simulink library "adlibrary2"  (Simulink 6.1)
undefined symbols (not defined in the file or in its folder): adlibrary2, ADM, Bit, Black, Box, d2sram_config, DDR, ddr32_config, ddr32xp_config, Generation, II, Inactive, Location, Lower, SDRAM, Simulation, Subsystem, Width, xbsIndex_r3, XPL, XRC, XRM, zbt32_config, zbt64_config, zbtXRC4_config
libraries: xbsIndex_r3 x786
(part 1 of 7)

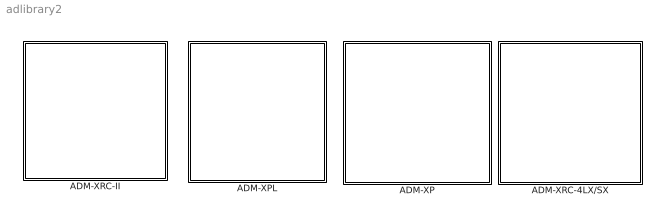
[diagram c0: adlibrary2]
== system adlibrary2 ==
  ADM-XP : Subsystem
  ADM-XPL : Subsystem
  ADM-XRC-4LX/SX : Subsystem  AncestorBlock=adlibrary2/ADM-XRC-II
  ADM-XRC-II : Subsystem

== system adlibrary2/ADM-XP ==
  DDR SDRAM 0 : Subsystem  mask{memsize=1}
      mask prompts: memsize "Simulation RAM Size (Mb)"
  DDR SDRAM 1 : Subsystem  mask{memsize=1}
      mask prompts: memsize "Simulation RAM Size (Mb)"
  DDRII SRAM 0 : Subsystem
  DDRII SRAM 1 : Subsystem
  DDRII SRAM 2 : Subsystem
  DDRII SRAM 3 : Subsystem
  XPL 32 Bit Interface : Subsystem  mask{program='load myprogram.txt', clock_ratio=1.5}
      mask prompts: program "Local Bus Script Program"; clock_ratio "Clock Ratio"
  XPL 64 Bit Interface : Subsystem  mask{program='load myprogram.txt', clock_ratio=1.5}
      mask prompts: program "Local Bus Script Program"; clock_ratio "Clock Ratio"

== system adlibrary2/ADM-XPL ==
  DDR SDRAM : Subsystem  mask{memsize=1}
      mask prompts: memsize "Simulation RAM Size (Mb)"
  XPL 32 Bit Interface : Subsystem  mask{program='load myprogram.txt', clock_ratio=1.5}
      mask prompts: program "Local Bus Script Program"; clock_ratio "Clock Ratio"
  XPL 64 Bit Interface : Subsystem  mask{program='load myprogram.txt', clock_ratio=1.5}
      mask prompts: program "Local Bus Script Program"; clock_ratio "Clock Ratio"
  ZBT SRAM 64 : Subsystem

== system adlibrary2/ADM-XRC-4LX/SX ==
  PLX 32 Bit Interface : Subsystem  mask{program='load myprogram.txt', clock_ratio=1.5}
      mask prompts: program "Local Bus Script Program"; clock_ratio "Clock Ratio"
  ZBT SRAM 0 : Subsystem
  ZBT SRAM 1 : Subsystem
  ZBT SRAM 2 : Subsystem
  ZBT SRAM 3 : Subsystem
  ZBT SRAM 4 : Subsystem
  ZBT SRAM 5 : Subsystem

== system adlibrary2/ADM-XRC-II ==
  PLX 32 Bit Interface : Subsystem  mask{program='load myprogram.txt', clock_ratio=1.5}
      mask prompts: program "Local Bus Script Program"; clock_ratio "Clock Ratio"
  "XRM DDR SDRAM " : Subsystem  mask{memsize=1}
      mask prompts: memsize "Simulation RAM Size (Mb)"
  ZBT SRAM 0 : Subsystem
  ZBT SRAM 1 : Subsystem
  ZBT SRAM 2 : Subsystem
  ZBT SRAM 3 : Subsystem
  ZBT SRAM 4 : Subsystem
  ZBT SRAM 5 : Subsystem

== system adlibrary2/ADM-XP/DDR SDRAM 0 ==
  cache_data_in : Inport  Port=1  LatchInput=off
  cache_addr : Inport  Port=2  LatchInput=off
  cache_write : Inport  Port=3  LatchInput=off
  ddr_page : Inport  Port=4  LatchInput=off
  ddr_addr : Inport  Port=5  LatchInput=off
  ddr_read : Inport  Port=6  LatchInput=off
  ddr_write : Inport  Port=7  LatchInput=off
  adlocb_in : Inport  Port=8  LatchInput=off
  Constant : xbsIndex_r3/Constant  const=0  equ=P=C  arith_type=Unsigned  n_bits=66  bin_pt=0  opselect=C  inp2=PCIN>>17  opr=+  inp1=P  carry=CIN  iostate=0  explicit_period=on  period=1  dbl_ovrd=off
  Convert : xbsIndex_r3/Convert  arith_type=Unsigned  n_bits=66  bin_pt=0  quantization=Truncate  overflow=Wrap  latency=0  explicit_period=on  period=1  dbl_ovrd=off  show_param=off  inserted_by_tool=off  pipeline=off
  DDR SDRAM 32Bit Generation : Subsystem  AncestorBlock=adlibrary2/ADM-XPL/DDR SDRAM /DDR SDRAM 32Bit Generation
  DDR SDRAM 32bit Simulation : Subsystem  mask{memsize=memsize}
      mask prompts: memsize "Simulation Ram Size (Mb)"
  Simulation Multiplexer : xbsIndex_r3/Simulation Multiplexer  sim_sel=1  hw_sel=2
  Simulation Multiplexer1 : xbsIndex_r3/Simulation Multiplexer  sim_sel=1  hw_sel=2
  Simulation Multiplexer2 : xbsIndex_r3/Simulation Multiplexer  sim_sel=1  hw_sel=2
  cache_data_out : Outport
  ddr_busy : Outport  Port=2
  adlocb_out : Outport  Port=3
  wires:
  cache_data_in/1 -> DDR SDRAM 32bit Simulation/1(cache_data_in), DDR SDRAM 32Bit Generation/1(cache_data_in)
  cache_addr/1 -> DDR SDRAM 32bit Simulation/2(cache_addr), DDR SDRAM 32Bit Generation/2(cache_addr)
  cache_write/1 -> DDR SDRAM 32bit Simulation/3(cache_write), DDR SDRAM 32Bit Generation/3(cache_write)
  ddr_page/1 -> DDR SDRAM 32bit Simulation/4(ddr_page), DDR SDRAM 32Bit Generation/4(ddr_page)
  ddr_addr/1 -> DDR SDRAM 32bit Simulation/5(ddr_addr), DDR SDRAM 32Bit Generation/5(ddr_addr)
  ddr_read/1 -> DDR SDRAM 32bit Simulation/6(ddr_read), DDR SDRAM 32Bit Generation/6(ddr_read)
  ddr_write/1 -> DDR SDRAM 32bit Simulation/7(ddr_write), DDR SDRAM 32Bit Generation/7(ddr_write)
  Simulation Multiplexer/1 -> cache_data_out/1
  Simulation Multiplexer1/1 -> ddr_busy/1
  Simulation Multiplexer2/1 -> adlocb_out/1
  DDR SDRAM 32bit Simulation/2(ddr_busy) -> Simulation Multiplexer1/1
  DDR SDRAM 32bit Simulation/1(cache_data_out) -> Simulation Multiplexer/1
  DDR SDRAM 32Bit Generation/1(cache_data_out) -> Simulation Multiplexer/2
  DDR SDRAM 32Bit Generation/2(ddr_busy) -> Simulation Multiplexer1/2
  adlocb_in/1 -> DDR SDRAM 32Bit Generation/8(adlocb_in)
  Constant/1 -> Simulation Multiplexer2/1
  Convert/1 -> Simulation Multiplexer2/2
  DDR SDRAM 32Bit Generation/3(adlocb_out) -> Convert/1

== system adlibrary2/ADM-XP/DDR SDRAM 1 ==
  cache_data_in : Inport  Port=1  LatchInput=off
  cache_addr : Inport  Port=2  LatchInput=off
  cache_write : Inport  Port=3  LatchInput=off
  ddr_page : Inport  Port=4  LatchInput=off
  ddr_addr : Inport  Port=5  LatchInput=off
  ddr_read : Inport  Port=6  LatchInput=off
  ddr_write : Inport  Port=7  LatchInput=off
  adlocb_in : Inport  Port=8  LatchInput=off
  Constant : xbsIndex_r3/Constant  const=0  equ=P=C  arith_type=Unsigned  n_bits=66  bin_pt=0  opselect=C  inp2=PCIN>>17  opr=+  inp1=P  carry=CIN  iostate=0  explicit_period=on  period=1  dbl_ovrd=off
  Convert : xbsIndex_r3/Convert  arith_type=Unsigned  n_bits=66  bin_pt=0  quantization=Truncate  overflow=Wrap  latency=0  explicit_period=on  period=1  dbl_ovrd=off  show_param=off  inserted_by_tool=off  pipeline=off
  DDR SDRAM 32Bit Generation : Subsystem  AncestorBlock=adlibrary2/ADM-XPL/DDR SDRAM /DDR SDRAM 32Bit Generation
  DDR SDRAM 32bit Simulation : Subsystem  mask{memsize=memsize}
      mask prompts: memsize "Simulation Ram Size (Mb)"
  Simulation Multiplexer : xbsIndex_r3/Simulation Multiplexer  sim_sel=1  hw_sel=2
  Simulation Multiplexer1 : xbsIndex_r3/Simulation Multiplexer  sim_sel=1  hw_sel=2
  Simulation Multiplexer2 : xbsIndex_r3/Simulation Multiplexer  sim_sel=1  hw_sel=2
  cache_data_out : Outport
  ddr_busy : Outport  Port=2
  adlocb_out : Outport  Port=3
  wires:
  DDR SDRAM 32Bit Generation/3(adlocb_out) -> Convert/1
  Convert/1 -> Simulation Multiplexer2/2
  Constant/1 -> Simulation Multiplexer2/1
  adlocb_in/1 -> DDR SDRAM 32Bit Generation/8(adlocb_in)
  DDR SDRAM 32Bit Generation/2(ddr_busy) -> Simulation Multiplexer1/2
  DDR SDRAM 32Bit Generation/1(cache_data_out) -> Simulation Multiplexer/2
  DDR SDRAM 32bit Simulation/1(cache_data_out) -> Simulation Multiplexer/1
  DDR SDRAM 32bit Simulation/2(ddr_busy) -> Simulation Multiplexer1/1
  Simulation Multiplexer2/1 -> adlocb_out/1
  Simulation Multiplexer1/1 -> ddr_busy/1
  Simulation Multiplexer/1 -> cache_data_out/1
  ddr_write/1 -> DDR SDRAM 32Bit Generation/7(ddr_write), DDR SDRAM 32bit Simulation/7(ddr_write)
  ddr_read/1 -> DDR SDRAM 32Bit Generation/6(ddr_read), DDR SDRAM 32bit Simulation/6(ddr_read)
  ddr_addr/1 -> DDR SDRAM 32Bit Generation/5(ddr_addr), DDR SDRAM 32bit Simulation/5(ddr_addr)
  ddr_page/1 -> DDR SDRAM 32Bit Generation/4(ddr_page), DDR SDRAM 32bit Simulation/4(ddr_page)
  cache_write/1 -> DDR SDRAM 32Bit Generation/3(cache_write), DDR SDRAM 32bit Simulation/3(cache_write)
  cache_addr/1 -> DDR SDRAM 32Bit Generation/2(cache_addr), DDR SDRAM 32bit Simulation/2(cache_addr)
  cache_data_in/1 -> DDR SDRAM 32Bit Generation/1(cache_data_in), DDR SDRAM 32bit Simulation/1(cache_data_in)

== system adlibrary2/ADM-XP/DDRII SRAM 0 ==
  d : Inport  Port=1  LatchInput=off
  a : Inport  Port=2  LatchInput=off
  w : Inport  Port=3  LatchInput=off
  r : Inport  Port=4  LatchInput=off
  be : Inport  Port=5  LatchInput=off
  adlocb_in : Inport  Port=6  LatchInput=off
  Constant : xbsIndex_r3/Constant  const=0  equ=P=C  arith_type=Unsigned  n_bits=66  bin_pt=0  opselect=C  inp2=PCIN>>17  opr=+  inp1=P  carry=CIN  iostate=0  explicit_period=on  period=1  dbl_ovrd=off
  DDRII SRAM Generation : Subsystem
  DDRII SRAM Simulation : Subsystem
  Register : xbsIndex_r3/Register  init=0  reg_only_valid=off  explicit_period=on  period=1  rst=off  en=off  out_en=off  dbl_ovrd=off  show_param=off
  Register1 : xbsIndex_r3/Register  init=0  reg_only_valid=off  explicit_period=on  period=1  rst=off  en=off  out_en=off  dbl_ovrd=off  show_param=off
  Simulation Multiplexer : xbsIndex_r3/Simulation Multiplexer  sim_sel=1  hw_sel=2
  Simulation Multiplexer1 : xbsIndex_r3/Simulation Multiplexer  sim_sel=1  hw_sel=2
  Simulation Multiplexer2 : xbsIndex_r3/Simulation Multiplexer  sim_sel=1  hw_sel=2
  q : Outport
  qv : Outport  Port=2
  adlocb_out : Outport  Port=3
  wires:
  be/1 -> DDRII SRAM Generation/5(be), DDRII SRAM Simulation/5(be)
  r/1 -> DDRII SRAM Simulation/4(r), DDRII SRAM Generation/4(r)
  w/1 -> DDRII SRAM Generation/3(w), DDRII SRAM Simulation/3(w)
  a/1 -> DDRII SRAM Generation/2(a), DDRII SRAM Simulation/2(a)
  d/1 -> DDRII SRAM Generation/1(d), DDRII SRAM Simulation/1(d)
  DDRII SRAM Simulation/1(q) -> Simulation Multiplexer/1
  DDRII SRAM Generation/1(q) -> Simulation Multiplexer/2
  Simulation Multiplexer/1 -> Register/1
  DDRII SRAM Generation/2(qv) -> Simulation Multiplexer1/2
  DDRII SRAM Simulation/2(qv) -> Simulation Multiplexer1/1
  DDRII SRAM Generation/3(adlocb_out) -> Simulation Multiplexer2/2
  Constant/1 -> Simulation Multiplexer2/1
  Simulation Multiplexer2/1 -> adlocb_out/1
  adlocb_in/1 -> DDRII SRAM Generation/6(adlocb_in)
  Simulation Multiplexer1/1 -> Register1/1
  Register/1 -> q/1
  Register1/1 -> qv/1

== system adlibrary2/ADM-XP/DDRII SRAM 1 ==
  d : Inport  Port=1  LatchInput=off
  a : Inport  Port=2  LatchInput=off
  w : Inport  Port=3  LatchInput=off
  r : Inport  Port=4  LatchInput=off
  be : Inport  Port=5  LatchInput=off
  adlocb_in : Inport  Port=6  LatchInput=off
  Constant : xbsIndex_r3/Constant  const=0  equ=P=C  arith_type=Unsigned  n_bits=66  bin_pt=0  opselect=C  inp2=PCIN>>17  opr=+  inp1=P  carry=CIN  iostate=0  explicit_period=on  period=1  dbl_ovrd=off
  DDRII SRAM Generation : Subsystem
  DDRII SRAM Simulation : Subsystem
  Register : xbsIndex_r3/Register  init=0  reg_only_valid=off  explicit_period=on  period=1  rst=off  en=off  out_en=off  dbl_ovrd=off  show_param=off
  Register1 : xbsIndex_r3/Register  init=0  reg_only_valid=off  explicit_period=on  period=1  rst=off  en=off  out_en=off  dbl_ovrd=off  show_param=off
  Simulation Multiplexer : xbsIndex_r3/Simulation Multiplexer  sim_sel=1  hw_sel=2
  Simulation Multiplexer1 : xbsIndex_r3/Simulation Multiplexer  sim_sel=1  hw_sel=2
  Simulation Multiplexer2 : xbsIndex_r3/Simulation Multiplexer  sim_sel=1  hw_sel=2
  q : Outport
  qv : Outport  Port=2
  adlocb_out : Outport  Port=3
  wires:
  adlocb_in/1 -> DDRII SRAM Generation/6(adlocb_in)
  Simulation Multiplexer2/1 -> adlocb_out/1
  Constant/1 -> Simulation Multiplexer2/1
  DDRII SRAM Generation/3(adlocb_out) -> Simulation Multiplexer2/2
  DDRII SRAM Simulation/2(qv) -> Simulation Multiplexer1/1
  DDRII SRAM Generation/2(qv) -> Simulation Multiplexer1/2
  Simulation Multiplexer/1 -> Register/1
  DDRII SRAM Generation/1(q) -> Simulation Multiplexer/2
  DDRII SRAM Simulation/1(q) -> Simulation Multiplexer/1
  d/1 -> DDRII SRAM Simulation/1(d), DDRII SRAM Generation/1(d)
  a/1 -> DDRII SRAM Simulation/2(a), DDRII SRAM Generation/2(a)
  w/1 -> DDRII SRAM Simulation/3(w), DDRII SRAM Generation/3(w)
  r/1 -> DDRII SRAM Simulation/4(r), DDRII SRAM Generation/4(r)
  be/1 -> DDRII SRAM Simulation/5(be), DDRII SRAM Generation/5(be)
  Simulation Multiplexer1/1 -> Register1/1
  Register/1 -> q/1
  Register1/1 -> qv/1

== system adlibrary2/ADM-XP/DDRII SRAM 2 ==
  d : Inport  Port=1  LatchInput=off
  a : Inport  Port=2  LatchInput=off
  w : Inport  Port=3  LatchInput=off
  r : Inport  Port=4  LatchInput=off
  be : Inport  Port=5  LatchInput=off
  adlocb_in : Inport  Port=6  LatchInput=off
  Constant : xbsIndex_r3/Constant  const=0  equ=P=C  arith_type=Unsigned  n_bits=66  bin_pt=0  opselect=C  inp2=PCIN>>17  opr=+  inp1=P  carry=CIN  iostate=0  explicit_period=on  period=1  dbl_ovrd=off
  DDRII SRAM Generation : Subsystem
  DDRII SRAM Simulation : Subsystem
  Register : xbsIndex_r3/Register  init=0  reg_only_valid=off  explicit_period=on  period=1  rst=off  en=off  out_en=off  dbl_ovrd=off  show_param=off
  Register1 : xbsIndex_r3/Register  init=0  reg_only_valid=off  explicit_period=on  period=1  rst=off  en=off  out_en=off  dbl_ovrd=off  show_param=off
  Simulation Multiplexer : xbsIndex_r3/Simulation Multiplexer  sim_sel=1  hw_sel=2
  Simulation Multiplexer1 : xbsIndex_r3/Simulation Multiplexer  sim_sel=1  hw_sel=2
  Simulation Multiplexer2 : xbsIndex_r3/Simulation Multiplexer  sim_sel=1  hw_sel=2
  q : Outport
  qv : Outport  Port=2
  adlocb_out : Outport  Port=3
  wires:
  adlocb_in/1 -> DDRII SRAM Generation/6(adlocb_in)
  Simulation Multiplexer2/1 -> adlocb_out/1
  Constant/1 -> Simulation Multiplexer2/1
  DDRII SRAM Generation/3(adlocb_out) -> Simulation Multiplexer2/2
  DDRII SRAM Simulation/2(qv) -> Simulation Multiplexer1/1
  DDRII SRAM Generation/2(qv) -> Simulation Multiplexer1/2
  Simulation Multiplexer/1 -> Register/1
  DDRII SRAM Generation/1(q) -> Simulation Multiplexer/2
  DDRII SRAM Simulation/1(q) -> Simulation Multiplexer/1
  d/1 -> DDRII SRAM Simulation/1(d), DDRII SRAM Generation/1(d)
  a/1 -> DDRII SRAM Simulation/2(a), DDRII SRAM Generation/2(a)
  w/1 -> DDRII SRAM Simulation/3(w), DDRII SRAM Generation/3(w)
  r/1 -> DDRII SRAM Simulation/4(r), DDRII SRAM Generation/4(r)
  be/1 -> DDRII SRAM Simulation/5(be), DDRII SRAM Generation/5(be)
  Simulation Multiplexer1/1 -> Register1/1
  Register/1 -> q/1
  Register1/1 -> qv/1

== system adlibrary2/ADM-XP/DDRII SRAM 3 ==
  d : Inport  Port=1  LatchInput=off
  a : Inport  Port=2  LatchInput=off
  w : Inport  Port=3  LatchInput=off
  r : Inport  Port=4  LatchInput=off
  be : Inport  Port=5  LatchInput=off
  adlocb_in : Inport  Port=6  LatchInput=off
  Constant : xbsIndex_r3/Constant  const=0  equ=P=C  arith_type=Unsigned  n_bits=66  bin_pt=0  opselect=C  inp2=PCIN>>17  opr=+  inp1=P  carry=CIN  iostate=0  explicit_period=on  period=1  dbl_ovrd=off
  DDRII SRAM Generation : Subsystem
  DDRII SRAM Simulation : Subsystem
  Register : xbsIndex_r3/Register  init=0  reg_only_valid=off  explicit_period=on  period=1  rst=off  en=off  out_en=off  dbl_ovrd=off  show_param=off
  Register1 : xbsIndex_r3/Register  init=0  reg_only_valid=off  explicit_period=on  period=1  rst=off  en=off  out_en=off  dbl_ovrd=off  show_param=off
  Simulation Multiplexer : xbsIndex_r3/Simulation Multiplexer  sim_sel=1  hw_sel=2
  Simulation Multiplexer1 : xbsIndex_r3/Simulation Multiplexer  sim_sel=1  hw_sel=2
  Simulation Multiplexer2 : xbsIndex_r3/Simulation Multiplexer  sim_sel=1  hw_sel=2
  q : Outport
  qv : Outport  Port=2
  adlocb_out : Outport  Port=3
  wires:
  adlocb_in/1 -> DDRII SRAM Generation/6(adlocb_in)
  Simulation Multiplexer2/1 -> adlocb_out/1
  Constant/1 -> Simulation Multiplexer2/1
  DDRII SRAM Generation/3(adlocb_out) -> Simulation Multiplexer2/2
  DDRII SRAM Simulation/2(qv) -> Simulation Multiplexer1/1
  DDRII SRAM Generation/2(read_pending) -> Simulation Multiplexer1/2
  Simulation Multiplexer/1 -> Register/1
  DDRII SRAM Generation/1(q) -> Simulation Multiplexer/2
  DDRII SRAM Simulation/1(q) -> Simulation Multiplexer/1
  d/1 -> DDRII SRAM Simulation/1(d), DDRII SRAM Generation/1(d)
  a/1 -> DDRII SRAM Simulation/2(a), DDRII SRAM Generation/2(a)
  w/1 -> DDRII SRAM Simulation/3(w), DDRII SRAM Generation/3(w)
  r/1 -> DDRII SRAM Simulation/4(r), DDRII SRAM Generation/4(r)
  be/1 -> DDRII SRAM Simulation/5(be), DDRII SRAM Generation/5(be)
  Simulation Multiplexer1/1 -> Register1/1
  Register/1 -> q/1
  Register1/1 -> qv/1

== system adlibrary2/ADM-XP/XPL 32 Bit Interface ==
  Data_Read : Inport  Port=1  LatchInput=off
  Ack : Inport  Port=2  LatchInput=off
  Status : Inport  Port=3  LatchInput=off
  Read IFIFO : Inport  Port=4  LatchInput=off
  Write OFIFO : Inport  Port=5  LatchInput=off
  OFIFO_Data : Inport  Port=6  LatchInput=off
  ADLOCB_IN : Inport  Port=7  LatchInput=off
  Constant : xbsIndex_r3/Constant  const=0  equ=P=C  arith_type=Unsigned  n_bits=66  bin_pt=0  opselect=C  inp2=PCIN>>17  opr=+  inp1=P  carry=CIN  iostate=0  explicit_period=on  period=1  dbl_ovrd=off
  Convert : xbsIndex_r3/Convert  arith_type=Unsigned  n_bits=66  bin_pt=0  quantization=Truncate  overflow=Wrap  latency=0  explicit_period=on  period=1  dbl_ovrd=off  show_param=off  inserted_by_tool=off  pipeline=off
  Simulation Multiplexer{,1..8,10} (10 alike) : xbsIndex_r3/Simulation Multiplexer  sim_sel=1  hw_sel=2
  XPL 32Bit Generation : Subsystem
  XPL 32Bit Simulation : Subsystem  mask{program=program, clock_ratio=clock_ratio}
      mask prompts: program "Local Bus Script Program"; clock_ratio "Clock Ratio"
  Data_Write : Outport
  Addr : Outport  Port=2
  BE : Outport  Port=3
  Write : Outport  Port=4
  Read : Outport  Port=5
  Control : Outport  Port=6
  IFIFO_Data : Outport  Port=7
  IFIFO_Empty : Outport  Port=8
  OFIFO_Full : Outport  Port=9
  ADLOCB_OUT : Outport  Port=10
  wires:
  ADLOCB_IN/1 -> XPL 32Bit Generation/7(adlocb_in)
  XPL 32Bit Generation/10(adlocb_out) -> Convert/1
  Convert/1 -> Simulation Multiplexer10/2
  Constant/1 -> Simulation Multiplexer10/1
  Simulation Multiplexer10/1 -> ADLOCB_OUT/1
  XPL 32Bit Generation/3(BE) -> Simulation Multiplexer1/2
  XPL 32Bit Simulation/3(BE) -> Simulation Multiplexer1/1
  XPL 32Bit Simulation/2(Addr) -> Simulation Multiplexer8/1
  Simulation Multiplexer8/1 -> Addr/1
  XPL 32Bit Simulation/4(Write) -> Simulation Multiplexer2/1
  XPL 32Bit Simulation/5(Read) -> Simulation Multiplexer3/1
  XPL 32Bit Simulation/6(Control) -> Simulation Multiplexer4/1
  XPL 32Bit Simulation/7(IFIFO_Data) -> Simulation Multiplexer5/1
  XPL 32Bit Simulation/8(IFIFO_Empty) -> Simulation Multiplexer6/1
  Simulation Multiplexer/1 -> Data_Write/1
  Simulation Multiplexer1/1 -> BE/1
  Simulation Multiplexer2/1 -> Write/1
  Simulation Multiplexer3/1 -> Read/1
  Simulation Multiplexer4/1 -> Control/1
  Simulation Multiplexer5/1 -> IFIFO_Data/1
  Simulation Multiplexer6/1 -> IFIFO_Empty/1
  Simulation Multiplexer7/1 -> OFIFO_Full/1
  XPL 32Bit Generation/9(OFIFO_Full) -> Simulation Multiplexer7/2
  XPL 32Bit Generation/8(IFIFO_Empty) -> Simulation Multiplexer6/2
  XPL 32Bit Generation/7(IFIFO_Data) -> Simulation Multiplexer5/2
  XPL 32Bit Generation/6(Control) -> Simulation Multiplexer4/2
  XPL 32Bit Generation/5(Read) -> Simulation Multiplexer3/2
  XPL 32Bit Generation/4(Write) -> Simulation Multiplexer2/2
  XPL 32Bit Generation/2(Addr) -> Simulation Multiplexer8/2
  XPL 32Bit Generation/1(Data_Write) -> Simulation Multiplexer/2
  XPL 32Bit Simulation/1(Data_Write) -> Simulation Multiplexer/1
  XPL 32Bit Simulation/9(OFIFO_Full) -> Simulation Multiplexer7/1
  Data_Read/1 -> XPL 32Bit Simulation/1(Data_Read), XPL 32Bit Generation/1(Data_Read)
  Ack/1 -> XPL 32Bit Simulation/2(Ack), XPL 32Bit Generation/2(Ack)
  Status/1 -> XPL 32Bit Simulation/3(Status), XPL 32Bit Generation/3(Status)
  Read IFIFO/1 -> XPL 32Bit Simulation/4(Read IFIFO), XPL 32Bit Generation/4(Read IFIFO)
  Write OFIFO/1 -> XPL 32Bit Simulation/5(Write OFIFO), XPL 32Bit Generation/5(Write OFIFO)
  OFIFO_Data/1 -> XPL 32Bit Simulation/6(OFIFO_Data), XPL 32Bit Generation/6(OFIFO_Data)

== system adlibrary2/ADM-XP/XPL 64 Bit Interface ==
  Data_Read : Inport  Port=1  LatchInput=off
  Ack : Inport  Port=2  LatchInput=off
  Status : Inport  Port=3  LatchInput=off
  Read IFIFO : Inport  Port=4  LatchInput=off
  Write OFIFO : Inport  Port=5  LatchInput=off
  OFIFO_Data : Inport  Port=6  LatchInput=off
  ADLOCB_IN : Inport  Port=7  LatchInput=off
  Constant : xbsIndex_r3/Constant  const=0  equ=P=C  arith_type=Unsigned  n_bits=66  bin_pt=0  opselect=C  inp2=PCIN>>17  opr=+  inp1=P  carry=CIN  iostate=0  explicit_period=on  period=1  dbl_ovrd=off
  Convert : xbsIndex_r3/Convert  arith_type=Unsigned  n_bits=66  bin_pt=0  quantization=Truncate  overflow=Wrap  latency=0  explicit_period=on  period=1  dbl_ovrd=off  show_param=off  inserted_by_tool=off  pipeline=off
  Simulation Multiplexer{,1..9} (10 alike) : xbsIndex_r3/Simulation Multiplexer  sim_sel=1  hw_sel=2
  XPL 64Bit Generation : Subsystem
  XPL 64Bit Simulation : Subsystem  mask{program=program, clock_ratio=clock_ratio}
      mask prompts: program "Local Bus Script Program"; clock_ratio "Clock Ratio"
  Data_Write : Outport
  Addr : Outport  Port=2
  BE : Outport  Port=3
  Write : Outport  Port=4
  Read : Outport  Port=5
  Control : Outport  Port=6
  IFIFO_Data : Outport  Port=7
  IFIFO_Empty : Outport  Port=8
  OFIFO_Full : Outport  Port=9
  ADLOCB_OUT : Outport  Port=10
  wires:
  XPL 64Bit Generation/10(adlocb_out) -> Convert/1
  Convert/1 -> Simulation Multiplexer9/2
  Constant/1 -> Simulation Multiplexer9/1
  ADLOCB_IN/1 -> XPL 64Bit Generation/7(adlocb_in)
  Simulation Multiplexer9/1 -> ADLOCB_OUT/1
  XPL 64Bit Simulation/3(BE) -> Simulation Multiplexer8/1
  XPL 64Bit Generation/3(BE) -> Simulation Multiplexer8/2
  Simulation Multiplexer8/1 -> BE/1
  OFIFO_Data/1 -> XPL 64Bit Generation/6(OFIFO_Data), XPL 64Bit Simulation/6(OFIFO_Data)
  Write OFIFO/1 -> XPL 64Bit Generation/5(Write OFIFO), XPL 64Bit Simulation/5(Write OFIFO)
  Read IFIFO/1 -> XPL 64Bit Generation/4(Read IFIFO), XPL 64Bit Simulation/4(Read IFIFO)
  Status/1 -> XPL 64Bit Generation/3(Status), XPL 64Bit Simulation/3(Status)
  Ack/1 -> XPL 64Bit Generation/2(Ack), XPL 64Bit Simulation/2(Ack)
  Data_Read/1 -> XPL 64Bit Generation/1(Data_Read), XPL 64Bit Simulation/1(Data_Read)
  XPL 64Bit Simulation/9(OFIFO_Full) -> Simulation Multiplexer7/1
  XPL 64Bit Simulation/8(IFIFO_Empty) -> Simulation Multiplexer6/1
  XPL 64Bit Simulation/7(IFIFO_Data) -> Simulation Multiplexer5/1
  XPL 64Bit Simulation/6(Control) -> Simulation Multiplexer4/1
  XPL 64Bit Simulation/5(Read) -> Simulation Multiplexer3/1
  XPL 64Bit Simulation/4(Write) -> Simulation Multiplexer2/1
  XPL 64Bit Simulation/2(Addr) -> Simulation Multiplexer1/1
  XPL 64Bit Simulation/1(Data_Write) -> Simulation Multiplexer/1
  XPL 64Bit Generation/1(Data_Write) -> Simulation Multiplexer/2
  XPL 64Bit Generation/2(Addr) -> Simulation Multiplexer1/2
  XPL 64Bit Generation/4(Write) -> Simulation Multiplexer2/2
  XPL 64Bit Generation/5(Read) -> Simulation Multiplexer3/2
  XPL 64Bit Generation/6(Control) -> Simulation Multiplexer4/2
  XPL 64Bit Generation/7(IFIFO_Data) -> Simulation Multiplexer5/2
  XPL 64Bit Generation/8(IFIFO_Empty) -> Simulation Multiplexer6/2
  XPL 64Bit Generation/9(OFIFO_Full) -> Simulation Multiplexer7/2
  Simulation Multiplexer7/1 -> OFIFO_Full/1
  Simulation Multiplexer6/1 -> IFIFO_Empty/1
  Simulation Multiplexer5/1 -> IFIFO_Data/1
  Simulation Multiplexer4/1 -> Control/1
  Simulation Multiplexer3/1 -> Read/1
  Simulation Multiplexer2/1 -> Write/1
  Simulation Multiplexer1/1 -> Addr/1
  Simulation Multiplexer/1 -> Data_Write/1

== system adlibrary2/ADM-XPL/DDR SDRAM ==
  cache_data_in : Inport  Port=1  LatchInput=off
  cache_addr : Inport  Port=2  LatchInput=off
  cache_write : Inport  Port=3  LatchInput=off
  ddr_page : Inport  Port=4  LatchInput=off
  ddr_addr : Inport  Port=5  LatchInput=off
  ddr_read : Inport  Port=6  LatchInput=off
  ddr_write : Inport  Port=7  LatchInput=off
  adlocb_in : Inport  Port=8  LatchInput=off
  Constant : xbsIndex_r3/Constant  const=0  equ=P=C  arith_type=Unsigned  n_bits=66  bin_pt=0  opselect=C  inp2=PCIN>>17  opr=+  inp1=P  carry=CIN  iostate=0  explicit_period=on  period=1  dbl_ovrd=off
  Convert : xbsIndex_r3/Convert  arith_type=Unsigned  n_bits=66  bin_pt=0  quantization=Truncate  overflow=Wrap  latency=0  explicit_period=on  period=1  dbl_ovrd=off  show_param=off  inserted_by_tool=off  pipeline=off
  DDR SDRAM 32Bit Generation : Subsystem  AncestorBlock=adlibrary2/ADM-XPL/DDR SDRAM /DDR SDRAM 32Bit Generation
  DDR SDRAM 32bit Simulation : Subsystem  mask{memsize=memsize}
      mask prompts: memsize "Simulation Ram Size (Mb)"
  Simulation Multiplexer : xbsIndex_r3/Simulation Multiplexer  sim_sel=1  hw_sel=2
  Simulation Multiplexer1 : xbsIndex_r3/Simulation Multiplexer  sim_sel=1  hw_sel=2
  Simulation Multiplexer2 : xbsIndex_r3/Simulation Multiplexer  sim_sel=1  hw_sel=2
  cache_data_out : Outport
  ddr_busy : Outport  Port=2
  adlocb_out : Outport  Port=3
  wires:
  DDR SDRAM 32Bit Generation/3(adlocb_out) -> Convert/1
  Convert/1 -> Simulation Multiplexer2/2
  Constant/1 -> Simulation Multiplexer2/1
  adlocb_in/1 -> DDR SDRAM 32Bit Generation/8(adlocb_in)
  DDR SDRAM 32Bit Generation/2(ddr_busy) -> Simulation Multiplexer1/2
  DDR SDRAM 32Bit Generation/1(cache_data_out) -> Simulation Multiplexer/2
  DDR SDRAM 32bit Simulation/1(cache_data_out) -> Simulation Multiplexer/1
  DDR SDRAM 32bit Simulation/2(ddr_busy) -> Simulation Multiplexer1/1
  Simulation Multiplexer2/1 -> adlocb_out/1
  Simulation Multiplexer1/1 -> ddr_busy/1
  Simulation Multiplexer/1 -> cache_data_out/1
  ddr_write/1 -> DDR SDRAM 32Bit Generation/7(ddr_write), DDR SDRAM 32bit Simulation/7(ddr_write)
  ddr_read/1 -> DDR SDRAM 32Bit Generation/6(ddr_read), DDR SDRAM 32bit Simulation/6(ddr_read)
  ddr_addr/1 -> DDR SDRAM 32Bit Generation/5(ddr_addr), DDR SDRAM 32bit Simulation/5(ddr_addr)
  ddr_page/1 -> DDR SDRAM 32Bit Generation/4(ddr_page), DDR SDRAM 32bit Simulation/4(ddr_page)
  cache_write/1 -> DDR SDRAM 32Bit Generation/3(cache_write), DDR SDRAM 32bit Simulation/3(cache_write)
  cache_addr/1 -> DDR SDRAM 32Bit Generation/2(cache_addr), DDR SDRAM 32bit Simulation/2(cache_addr)
  cache_data_in/1 -> DDR SDRAM 32Bit Generation/1(cache_data_in), DDR SDRAM 32bit Simulation/1(cache_data_in)

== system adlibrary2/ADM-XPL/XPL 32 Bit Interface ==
  Data_Read : Inport  Port=1  LatchInput=off
  Ack : Inport  Port=2  LatchInput=off
  Status : Inport  Port=3  LatchInput=off
  Read IFIFO : Inport  Port=4  LatchInput=off
  Write OFIFO : Inport  Port=5  LatchInput=off
  OFIFO_Data : Inport  Port=6  LatchInput=off
  ADLOCB_IN : Inport  Port=7  LatchInput=off
  Constant : xbsIndex_r3/Constant  const=0  equ=P=C  arith_type=Unsigned  n_bits=66  bin_pt=0  opselect=C  inp2=PCIN>>17  opr=+  inp1=P  carry=CIN  iostate=0  explicit_period=on  period=1  dbl_ovrd=off
  Convert : xbsIndex_r3/Convert  arith_type=Unsigned  n_bits=66  bin_pt=0  quantization=Truncate  overflow=Wrap  latency=0  explicit_period=on  period=1  dbl_ovrd=off  show_param=off  inserted_by_tool=off  pipeline=off
  Simulation Multiplexer{,1..8,10} (10 alike) : xbsIndex_r3/Simulation Multiplexer  sim_sel=1  hw_sel=2
  XPL 32Bit Generation : Subsystem
  XPL 32Bit Simulation : Subsystem  mask{program=program, clock_ratio=clock_ratio}
      mask prompts: program "Local Bus Script Program"; clock_ratio "Clock Ratio"
  Data_Write : Outport
  Addr : Outport  Port=2
  BE : Outport  Port=3
  Write : Outport  Port=4
  Read : Outport  Port=5
  Control : Outport  Port=6
  IFIFO_Data : Outport  Port=7
  IFIFO_Empty : Outport  Port=8
  OFIFO_Full : Outport  Port=9
  ADLOCB_OUT : Outport  Port=10
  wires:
  OFIFO_Data/1 -> XPL 32Bit Generation/6(OFIFO_Data), XPL 32Bit Simulation/6(OFIFO_Data)
  Write OFIFO/1 -> XPL 32Bit Generation/5(Write OFIFO), XPL 32Bit Simulation/5(Write OFIFO)
  Read IFIFO/1 -> XPL 32Bit Generation/4(Read IFIFO), XPL 32Bit Simulation/4(Read IFIFO)
  Status/1 -> XPL 32Bit Generation/3(Status), XPL 32Bit Simulation/3(Status)
  Ack/1 -> XPL 32Bit Generation/2(Ack), XPL 32Bit Simulation/2(Ack)
  Data_Read/1 -> XPL 32Bit Generation/1(Data_Read), XPL 32Bit Simulation/1(Data_Read)
  XPL 32Bit Simulation/9(OFIFO_Full) -> Simulation Multiplexer7/1
  XPL 32Bit Simulation/1(Data_Write) -> Simulation Multiplexer/1
  XPL 32Bit Generation/1(Data_Write) -> Simulation Multiplexer/2
  XPL 32Bit Generation/2(Addr) -> Simulation Multiplexer8/2
  XPL 32Bit Generation/4(Write) -> Simulation Multiplexer2/2
  XPL 32Bit Generation/5(Read) -> Simulation Multiplexer3/2
  XPL 32Bit Generation/6(Control) -> Simulation Multiplexer4/2
  XPL 32Bit Generation/7(IFIFO_Data) -> Simulation Multiplexer5/2
  XPL 32Bit Generation/8(IFIFO_Empty) -> Simulation Multiplexer6/2
  XPL 32Bit Generation/9(OFIFO_Full) -> Simulation Multiplexer7/2
  Simulation Multiplexer7/1 -> OFIFO_Full/1
  Simulation Multiplexer6/1 -> IFIFO_Empty/1
  Simulation Multiplexer5/1 -> IFIFO_Data/1
  Simulation Multiplexer4/1 -> Control/1
  Simulation Multiplexer3/1 -> Read/1
  Simulation Multiplexer2/1 -> Write/1
  Simulation Multiplexer1/1 -> BE/1
  Simulation Multiplexer/1 -> Data_Write/1
  XPL 32Bit Simulation/8(IFIFO_Empty) -> Simulation Multiplexer6/1
  XPL 32Bit Simulation/7(IFIFO_Data) -> Simulation Multiplexer5/1
  XPL 32Bit Simulation/6(Control) -> Simulation Multiplexer4/1
  XPL 32Bit Simulation/5(Read) -> Simulation Multiplexer3/1
  XPL 32Bit Simulation/4(Write) -> Simulation Multiplexer2/1
  Simulation Multiplexer8/1 -> Addr/1
  XPL 32Bit Simulation/2(Addr) -> Simulation Multiplexer8/1
  XPL 32Bit Simulation/3(BE) -> Simulation Multiplexer1/1
  XPL 32Bit Generation/3(BE) -> Simulation Multiplexer1/2
  Simulation Multiplexer10/1 -> ADLOCB_OUT/1
  Constant/1 -> Simulation Multiplexer10/1
  Convert/1 -> Simulation Multiplexer10/2
  XPL 32Bit Generation/10(adlocb_out) -> Convert/1
  ADLOCB_IN/1 -> XPL 32Bit Generation/7(adlocb_in)

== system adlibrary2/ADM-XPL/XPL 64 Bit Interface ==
  Data_Read : Inport  Port=1  LatchInput=off
  Ack : Inport  Port=2  LatchInput=off
  Status : Inport  Port=3  LatchInput=off
  Read IFIFO : Inport  Port=4  LatchInput=off
  Write OFIFO : Inport  Port=5  LatchInput=off
  OFIFO_Data : Inport  Port=6  LatchInput=off
  ADLOCB_IN : Inport  Port=7  LatchInput=off
  Constant : xbsIndex_r3/Constant  const=0  equ=P=C  arith_type=Unsigned  n_bits=66  bin_pt=0  opselect=C  inp2=PCIN>>17  opr=+  inp1=P  carry=CIN  iostate=0  explicit_period=on  period=1  dbl_ovrd=off
  Convert : xbsIndex_r3/Convert  arith_type=Unsigned  n_bits=66  bin_pt=0  quantization=Truncate  overflow=Wrap  latency=0  explicit_period=on  period=1  dbl_ovrd=off  show_param=off  inserted_by_tool=off  pipeline=off
  Simulation Multiplexer{,1..9} (10 alike) : xbsIndex_r3/Simulation Multiplexer  sim_sel=1  hw_sel=2
  XPL 64Bit Generation : Subsystem
  XPL 64Bit Simulation : Subsystem  mask{program=program, clock_ratio=clock_ratio}
      mask prompts: program "Local Bus Script Program"; clock_ratio "Clock Ratio"
  Data_Write : Outport
  Addr : Outport  Port=2
  BE : Outport  Port=3
  Write : Outport  Port=4
  Read : Outport  Port=5
  Control : Outport  Port=6
  IFIFO_Data : Outport  Port=7
  IFIFO_Empty : Outport  Port=8
  OFIFO_Full : Outport  Port=9
  ADLOCB_OUT : Outport  Port=10
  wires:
  Simulation Multiplexer/1 -> Data_Write/1
  Simulation Multiplexer1/1 -> Addr/1
  Simulation Multiplexer2/1 -> Write/1
  Simulation Multiplexer3/1 -> Read/1
  Simulation Multiplexer4/1 -> Control/1
  Simulation Multiplexer5/1 -> IFIFO_Data/1
  Simulation Multiplexer6/1 -> IFIFO_Empty/1
  Simulation Multiplexer7/1 -> OFIFO_Full/1
  XPL 64Bit Generation/9(OFIFO_Full) -> Simulation Multiplexer7/2
  XPL 64Bit Generation/8(IFIFO_Empty) -> Simulation Multiplexer6/2
  XPL 64Bit Generation/7(IFIFO_Data) -> Simulation Multiplexer5/2
  XPL 64Bit Generation/6(Control) -> Simulation Multiplexer4/2
  XPL 64Bit Generation/5(Read) -> Simulation Multiplexer3/2
  XPL 64Bit Generation/4(Write) -> Simulation Multiplexer2/2
  XPL 64Bit Generation/2(Addr) -> Simulation Multiplexer1/2
  XPL 64Bit Generation/1(Data_Write) -> Simulation Multiplexer/2
  XPL 64Bit Simulation/1(Data_Write) -> Simulation Multiplexer/1
  XPL 64Bit Simulation/2(Addr) -> Simulation Multiplexer1/1
  XPL 64Bit Simulation/4(Write) -> Simulation Multiplexer2/1
  XPL 64Bit Simulation/5(Read) -> Simulation Multiplexer3/1
  XPL 64Bit Simulation/6(Control) -> Simulation Multiplexer4/1
  XPL 64Bit Simulation/7(IFIFO_Data) -> Simulation Multiplexer5/1
  XPL 64Bit Simulation/8(IFIFO_Empty) -> Simulation Multiplexer6/1
  XPL 64Bit Simulation/9(OFIFO_Full) -> Simulation Multiplexer7/1
  Data_Read/1 -> XPL 64Bit Simulation/1(Data_Read), XPL 64Bit Generation/1(Data_Read)
  Ack/1 -> XPL 64Bit Simulation/2(Ack), XPL 64Bit Generation/2(Ack)
  Status/1 -> XPL 64Bit Simulation/3(Status), XPL 64Bit Generation/3(Status)
  Read IFIFO/1 -> XPL 64Bit Simulation/4(Read IFIFO), XPL 64Bit Generation/4(Read IFIFO)
  Write OFIFO/1 -> XPL 64Bit Simulation/5(Write OFIFO), XPL 64Bit Generation/5(Write OFIFO)
  OFIFO_Data/1 -> XPL 64Bit Simulation/6(OFIFO_Data), XPL 64Bit Generation/6(OFIFO_Data)
  Simulation Multiplexer8/1 -> BE/1
  XPL 64Bit Generation/3(BE) -> Simulation Multiplexer8/2
  XPL 64Bit Simulation/3(BE) -> Simulation Multiplexer8/1
  Simulation Multiplexer9/1 -> ADLOCB_OUT/1
  ADLOCB_IN/1 -> XPL 64Bit Generation/7(adlocb_in)
  Constant/1 -> Simulation Multiplexer9/1
  Convert/1 -> Simulation Multiplexer9/2
  XPL 64Bit Generation/10(adlocb_out) -> Convert/1

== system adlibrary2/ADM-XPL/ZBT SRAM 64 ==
  d : Inport  Port=1  LatchInput=off
  a : Inport  Port=2  LatchInput=off
  w : Inport  Port=3  LatchInput=off
  r : Inport  Port=4  LatchInput=off
  be : Inport  Port=5  LatchInput=off
  adlocb_in : Inport  Port=6  LatchInput=off
  Constant : xbsIndex_r3/Constant  const=0  equ=P=C  arith_type=Unsigned  n_bits=66  bin_pt=0  opselect=C  inp2=PCIN>>17  opr=+  inp1=P  carry=CIN  iostate=0  explicit_period=on  period=1  dbl_ovrd=off
  Simulation Multiplexer : xbsIndex_r3/Simulation Multiplexer  sim_sel=1  hw_sel=2
  Simulation Multiplexer1 : xbsIndex_r3/Simulation Multiplexer  sim_sel=1  hw_sel=2
  Simulation Multiplexer2 : xbsIndex_r3/Simulation Multiplexer  sim_sel=1  hw_sel=2
  ZBT SRAM 64Bit Generation : Subsystem
  ZBT SRAM 64bit Simulation : Subsystem
  q : Outport
  qv : Outport  Port=2
  adlocb_out : Outport  Port=3
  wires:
  Simulation Multiplexer/1 -> q/1
  ZBT SRAM 64Bit Generation/1(q) -> Simulation Multiplexer/2
  ZBT SRAM 64bit Simulation/1(q) -> Simulation Multiplexer/1
  d/1 -> ZBT SRAM 64bit Simulation/1(d), ZBT SRAM 64Bit Generation/1(d)
  a/1 -> ZBT SRAM 64bit Simulation/2(a), ZBT SRAM 64Bit Generation/2(a)
  w/1 -> ZBT SRAM 64bit Simulation/3(w), ZBT SRAM 64Bit Generation/3(w)
  Simulation Multiplexer1/1 -> qv/1
  r/1 -> ZBT SRAM 64bit Simulation/4(r), ZBT SRAM 64Bit Generation/4(r)
  ZBT SRAM 64bit Simulation/2(qv) -> Simulation Multiplexer1/1
  ZBT SRAM 64Bit Generation/2(qv) -> Simulation Multiplexer1/2
  be/1 -> ZBT SRAM 64bit Simulation/5(be), ZBT SRAM 64Bit Generation/5(be)
  Simulation Multiplexer2/1 -> adlocb_out/1
  ZBT SRAM 64Bit Generation/3(adlocb_out) -> Simulation Multiplexer2/2
  Constant/1 -> Simulation Multiplexer2/1
  adlocb_in/1 -> ZBT SRAM 64Bit Generation/6(adlocb_in)

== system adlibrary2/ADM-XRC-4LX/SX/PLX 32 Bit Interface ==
  Data_Read : Inport  Port=1  LatchInput=off
  Ack : Inport  Port=2  LatchInput=off
  Status : Inport  Port=3  LatchInput=off
  Read IFIFO : Inport  Port=4  LatchInput=off
  Write OFIFO : Inport  Port=5  LatchInput=off
  OFIFO_Data : Inport  Port=6  LatchInput=off
  ADLOCB_IN : Inport  Port=7  LatchInput=off
  Constant : xbsIndex_r3/Constant  const=0  equ=P=C  arith_type=Unsigned  n_bits=34  bin_pt=0  opselect=C  inp2=PCIN>>17  opr=+  inp1=P  carry=CIN  iostate=0  explicit_period=on  period=1  dbl_ovrd=off
  Convert : xbsIndex_r3/Convert  arith_type=Unsigned  n_bits=34  bin_pt=0  quantization=Truncate  overflow=Wrap  latency=0  explicit_period=on  period=1  dbl_ovrd=off  show_param=off  inserted_by_tool=off  pipeline=off
  PLX 32Bit Generation : Subsystem
  PLX 32Bit Simulation : Subsystem  mask{program=program, clock_ratio=clock_ratio}
      mask prompts: program "Local Bus Script Program"; clock_ratio "Clock Ratio"
  Simulation Multiplexer{,1..9} (10 alike) : xbsIndex_r3/Simulation Multiplexer  sim_sel=1  hw_sel=2
  Data_Write : Outport
  Addr : Outport  Port=2
  BE : Outport  Port=3
  Write : Outport  Port=4
  Read : Outport  Port=5
  Control : Outport  Port=6
  IFIFO_Data : Outport  Port=7
  IFIFO_Empty : Outport  Port=8
  OFIFO_Full : Outport  Port=9
  ADLOCB_OUT : Outport  Port=10
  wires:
  Data_Read/1 -> PLX 32Bit Generation/1(Data_Read), PLX 32Bit Simulation/1(Data_Read)
  Ack/1 -> PLX 32Bit Generation/2(Ack), PLX 32Bit Simulation/2(Ack)
  Status/1 -> PLX 32Bit Generation/3(Status), PLX 32Bit Simulation/3(Status)
  Read IFIFO/1 -> PLX 32Bit Generation/4(Read IFIFO), PLX 32Bit Simulation/4(Read IFIFO)
  Write OFIFO/1 -> PLX 32Bit Generation/5(Write OFIFO), PLX 32Bit Simulation/5(Write OFIFO)
  OFIFO_Data/1 -> PLX 32Bit Generation/6(OFIFO_Data), PLX 32Bit Simulation/6(OFIFO_Data)
  Simulation Multiplexer/1 -> Data_Write/1
  Simulation Multiplexer1/1 -> Addr/1
  Simulation Multiplexer2/1 -> Write/1
  Simulation Multiplexer3/1 -> Read/1
  Simulation Multiplexer4/1 -> Control/1
  Simulation Multiplexer5/1 -> IFIFO_Data/1
  Simulation Multiplexer6/1 -> IFIFO_Empty/1
  Simulation Multiplexer7/1 -> OFIFO_Full/1
  PLX 32Bit Generation/9(OFIFO_Full) -> Simulation Multiplexer7/2
  PLX 32Bit Generation/8(IFIFO_Empty) -> Simulation Multiplexer6/2
  PLX 32Bit Generation/7(IFIFO_Data) -> Simulation Multiplexer5/2
  PLX 32Bit Generation/6(Control) -> Simulation Multiplexer4/2
  PLX 32Bit Generation/5(Read) -> Simulation Multiplexer3/2
  PLX 32Bit Generation/4(Write) -> Simulation Multiplexer2/2
  PLX 32Bit Generation/2(Addr) -> Simulation Multiplexer1/2
  PLX 32Bit Generation/1(Data_Write) -> Simulation Multiplexer/2
  PLX 32Bit Simulation/1(Data_Write) -> Simulation Multiplexer/1
  PLX 32Bit Simulation/2(Addr) -> Simulation Multiplexer1/1
  PLX 32Bit Simulation/4(Write) -> Simulation Multiplexer2/1
  PLX 32Bit Simulation/5(Read) -> Simulation Multiplexer3/1
  PLX 32Bit Simulation/6(Control) -> Simulation Multiplexer4/1
  PLX 32Bit Simulation/7(IFIFO_Data) -> Simulation Multiplexer5/1
  PLX 32Bit Simulation/8(IFIFO_Empty) -> Simulation Multiplexer6/1
  PLX 32Bit Simulation/9(OFIFO_Full) -> Simulation Multiplexer7/1
  Simulation Multiplexer8/1 -> BE/1
  PLX 32Bit Generation/3(BE) -> Simulation Multiplexer8/2
  PLX 32Bit Simulation/3(BE) -> Simulation Multiplexer8/1
  Simulation Multiplexer9/1 -> ADLOCB_OUT/1
  PLX 32Bit Generation/10(ADLOCB_OUT) -> Convert/1
  ADLOCB_IN/1 -> PLX 32Bit Generation/7(ADLOCB_IN)
  Constant/1 -> Simulation Multiplexer9/1
  Convert/1 -> Simulation Multiplexer9/2

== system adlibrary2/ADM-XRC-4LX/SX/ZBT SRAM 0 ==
  d : Inport  Port=1  LatchInput=off
  a : Inport  Port=2  LatchInput=off
  w : Inport  Port=3  LatchInput=off
  r : Inport  Port=4  LatchInput=off
  be : Inport  Port=5  LatchInput=off
  adlocb_in : Inport  Port=6  LatchInput=off
  Constant : xbsIndex_r3/Constant  const=0  equ=P=C  arith_type=Unsigned  n_bits=34  bin_pt=0  opselect=C  inp2=PCIN>>17  opr=+  inp1=P  carry=CIN  iostate=0  explicit_period=on  period=1  dbl_ovrd=off
  Simulation Multiplexer : xbsIndex_r3/Simulation Multiplexer  sim_sel=1  hw_sel=2
  Simulation Multiplexer1 : xbsIndex_r3/Simulation Multiplexer  sim_sel=1  hw_sel=2
  Simulation Multiplexer2 : xbsIndex_r3/Simulation Multiplexer  sim_sel=1  hw_sel=2
  ZBT SRAM 32Bit Generation : Subsystem
  ZBT SRAM 32Bit Simulation : Subsystem
  q : Outport
  qv : Outport  Port=2
  adlocb_out : Outport  Port=3
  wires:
  r/1 -> ZBT SRAM 32Bit Generation/4(r), ZBT SRAM 32Bit Simulation/4(r)
  w/1 -> ZBT SRAM 32Bit Generation/3(w), ZBT SRAM 32Bit Simulation/3(w)
  a/1 -> ZBT SRAM 32Bit Generation/2(a), ZBT SRAM 32Bit Simulation/2(a)
  d/1 -> ZBT SRAM 32Bit Generation/1(d), ZBT SRAM 32Bit Simulation/1(d)
  ZBT SRAM 32Bit Simulation/2(qv) -> Simulation Multiplexer1/1
  ZBT SRAM 32Bit Simulation/1(q) -> Simulation Multiplexer/1
  ZBT SRAM 32Bit Generation/1(q) -> Simulation Multiplexer/2
  ZBT SRAM 32Bit Generation/2(qv) -> Simulation Multiplexer1/2
  Simulation Multiplexer1/1 -> qv/1
  Simulation Multiplexer/1 -> q/1
  be/1 -> ZBT SRAM 32Bit Simulation/5(be), ZBT SRAM 32Bit Generation/5(be)
  Simulation Multiplexer2/1 -> adlocb_out/1
  ZBT SRAM 32Bit Generation/3(adlocb_out) -> Simulation Multiplexer2/2
  adlocb_in/1 -> ZBT SRAM 32Bit Generation/6(adlocb_in)
  Constant/1 -> Simulation Multiplexer2/1

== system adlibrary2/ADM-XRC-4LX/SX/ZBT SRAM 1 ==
  d : Inport  Port=1  LatchInput=off
  a : Inport  Port=2  LatchInput=off
  w : Inport  Port=3  LatchInput=off
  r : Inport  Port=4  LatchInput=off
  be : Inport  Port=5  LatchInput=off
  adlocb_in : Inport  Port=6  LatchInput=off
  Constant : xbsIndex_r3/Constant  const=0  equ=P=C  arith_type=Unsigned  n_bits=34  bin_pt=0  opselect=C  inp2=PCIN>>17  opr=+  inp1=P  carry=CIN  iostate=0  explicit_period=on  period=1  dbl_ovrd=off
  Convert : xbsIndex_r3/Convert  arith_type=Unsigned  n_bits=34  bin_pt=0  quantization=Truncate  overflow=Wrap  latency=0  explicit_period=on  period=1  dbl_ovrd=off  show_param=off  inserted_by_tool=off  pipeline=off
  Simulation Multiplexer : xbsIndex_r3/Simulation Multiplexer  sim_sel=1  hw_sel=2
  Simulation Multiplexer1 : xbsIndex_r3/Simulation Multiplexer  sim_sel=1  hw_sel=2
  Simulation Multiplexer2 : xbsIndex_r3/Simulation Multiplexer  sim_sel=1  hw_sel=2
  ZBT SRAM 32Bit Generation : Subsystem
  ZBT SRAM 32Bit Simulation : Subsystem
  q : Outport
  qv : Outport  Port=2
  adlocb_out : Outport  Port=3
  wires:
  Constant/1 -> Simulation Multiplexer2/1
  adlocb_in/1 -> ZBT SRAM 32Bit Generation/6(adlocb_in)
  ZBT SRAM 32Bit Generation/3(adlocb_out) -> Convert/1
  Simulation Multiplexer2/1 -> adlocb_out/1
  be/1 -> ZBT SRAM 32Bit Generation/5(be), ZBT SRAM 32Bit Simulation/5(be)
  Simulation Multiplexer/1 -> q/1
  Simulation Multiplexer1/1 -> qv/1
  ZBT SRAM 32Bit Generation/2(qv) -> Simulation Multiplexer1/2
  ZBT SRAM 32Bit Generation/1(q) -> Simulation Multiplexer/2
  ZBT SRAM 32Bit Simulation/1(q) -> Simulation Multiplexer/1
  ZBT SRAM 32Bit Simulation/2(qv) -> Simulation Multiplexer1/1
  d/1 -> ZBT SRAM 32Bit Simulation/1(d), ZBT SRAM 32Bit Generation/1(d)
  a/1 -> ZBT SRAM 32Bit Simulation/2(a), ZBT SRAM 32Bit Generation/2(a)
  w/1 -> ZBT SRAM 32Bit Simulation/3(w), ZBT SRAM 32Bit Generation/3(w)
  r/1 -> ZBT SRAM 32Bit Simulation/4(r), ZBT SRAM 32Bit Generation/4(r)
  Convert/1 -> Simulation Multiplexer2/2

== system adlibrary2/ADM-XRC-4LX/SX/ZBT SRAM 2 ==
  d : Inport  Port=1  LatchInput=off
  a : Inport  Port=2  LatchInput=off
  w : Inport  Port=3  LatchInput=off
  r : Inport  Port=4  LatchInput=off
  be : Inport  Port=5  LatchInput=off
  adlocb_in : Inport  Port=6  LatchInput=off
  Constant : xbsIndex_r3/Constant  const=0  equ=P=C  arith_type=Unsigned  n_bits=34  bin_pt=0  opselect=C  inp2=PCIN>>17  opr=+  inp1=P  carry=CIN  iostate=0  explicit_period=on  period=1  dbl_ovrd=off
  Convert : xbsIndex_r3/Convert  arith_type=Unsigned  n_bits=34  bin_pt=0  quantization=Truncate  overflow=Wrap  latency=0  explicit_period=on  period=1  dbl_ovrd=off  show_param=off  inserted_by_tool=off  pipeline=off
  Simulation Multiplexer : xbsIndex_r3/Simulation Multiplexer  sim_sel=1  hw_sel=2
  Simulation Multiplexer1 : xbsIndex_r3/Simulation Multiplexer  sim_sel=1  hw_sel=2
  Simulation Multiplexer2 : xbsIndex_r3/Simulation Multiplexer  sim_sel=1  hw_sel=2
  ZBT SRAM 32Bit Generation : Subsystem
  ZBT SRAM 32Bit Simulation : Subsystem
  q : Outport
  qv : Outport  Port=2
  adlocb_out : Outport  Port=3
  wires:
  Constant/1 -> Simulation Multiplexer2/1
  adlocb_in/1 -> ZBT SRAM 32Bit Generation/6(adlocb_in)
  ZBT SRAM 32Bit Generation/3(adlocb_out) -> Convert/1
  Simulation Multiplexer2/1 -> adlocb_out/1
  be/1 -> ZBT SRAM 32Bit Generation/5(be), ZBT SRAM 32Bit Simulation/5(be)
  Simulation Multiplexer/1 -> q/1
  Simulation Multiplexer1/1 -> qv/1
  ZBT SRAM 32Bit Generation/2(qv) -> Simulation Multiplexer1/2
  ZBT SRAM 32Bit Generation/1(q) -> Simulation Multiplexer/2
  ZBT SRAM 32Bit Simulation/1(q) -> Simulation Multiplexer/1
  ZBT SRAM 32Bit Simulation/2(qv) -> Simulation Multiplexer1/1
  d/1 -> ZBT SRAM 32Bit Simulation/1(d), ZBT SRAM 32Bit Generation/1(d)
  a/1 -> ZBT SRAM 32Bit Simulation/2(a), ZBT SRAM 32Bit Generation/2(a)
  w/1 -> ZBT SRAM 32Bit Simulation/3(w), ZBT SRAM 32Bit Generation/3(w)
  r/1 -> ZBT SRAM 32Bit Simulation/4(r), ZBT SRAM 32Bit Generation/4(r)
  Convert/1 -> Simulation Multiplexer2/2

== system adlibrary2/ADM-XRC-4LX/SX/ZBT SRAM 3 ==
  d : Inport  Port=1  LatchInput=off
  a : Inport  Port=2  LatchInput=off
  w : Inport  Port=3  LatchInput=off
  r : Inport  Port=4  LatchInput=off
  be : Inport  Port=5  LatchInput=off
  adlocb_in : Inport  Port=6  LatchInput=off
  Constant : xbsIndex_r3/Constant  const=0  equ=P=C  arith_type=Unsigned  n_bits=34  bin_pt=0  opselect=C  inp2=PCIN>>17  opr=+  inp1=P  carry=CIN  iostate=0  explicit_period=on  period=1  dbl_ovrd=off
  Convert : xbsIndex_r3/Convert  arith_type=Unsigned  n_bits=34  bin_pt=0  quantization=Truncate  overflow=Wrap  latency=0  explicit_period=on  period=1  dbl_ovrd=off  show_param=off  inserted_by_tool=off  pipeline=off
  Simulation Multiplexer : xbsIndex_r3/Simulation Multiplexer  sim_sel=1  hw_sel=2
  Simulation Multiplexer1 : xbsIndex_r3/Simulation Multiplexer  sim_sel=1  hw_sel=2
  Simulation Multiplexer2 : xbsIndex_r3/Simulation Multiplexer  sim_sel=1  hw_sel=2
  ZBT SRAM 32Bit Generation : Subsystem
  ZBT SRAM 32Bit Simulation : Subsystem
  q : Outport
  qv : Outport  Port=2
  adlocb_out : Outport  Port=3
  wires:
  r/1 -> ZBT SRAM 32Bit Generation/4(r), ZBT SRAM 32Bit Simulation/4(r)
  w/1 -> ZBT SRAM 32Bit Generation/3(w), ZBT SRAM 32Bit Simulation/3(w)
  a/1 -> ZBT SRAM 32Bit Generation/2(a), ZBT SRAM 32Bit Simulation/2(a)
  d/1 -> ZBT SRAM 32Bit Generation/1(d), ZBT SRAM 32Bit Simulation/1(d)
  ZBT SRAM 32Bit Simulation/2(qv) -> Simulation Multiplexer1/1
  ZBT SRAM 32Bit Simulation/1(q) -> Simulation Multiplexer/1
  ZBT SRAM 32Bit Generation/1(q) -> Simulation Multiplexer/2
  ZBT SRAM 32Bit Generation/2(qv) -> Simulation Multiplexer1/2
  Simulation Multiplexer1/1 -> qv/1
  Simulation Multiplexer/1 -> q/1
  be/1 -> ZBT SRAM 32Bit Simulation/5(be), ZBT SRAM 32Bit Generation/5(be)
  Simulation Multiplexer2/1 -> adlocb_out/1
  ZBT SRAM 32Bit Generation/3(adlocb_out) -> Convert/1
  adlocb_in/1 -> ZBT SRAM 32Bit Generation/6(adlocb_in)
  Constant/1 -> Simulation Multiplexer2/1
  Convert/1 -> Simulation Multiplexer2/2

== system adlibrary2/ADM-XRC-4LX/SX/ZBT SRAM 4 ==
  d : Inport  Port=1  LatchInput=off
  a : Inport  Port=2  LatchInput=off
  w : Inport  Port=3  LatchInput=off
  r : Inport  Port=4  LatchInput=off
  be : Inport  Port=5  LatchInput=off
  adlocb_in : Inport  Port=6  LatchInput=off
  Constant : xbsIndex_r3/Constant  const=0  equ=P=C  arith_type=Unsigned  n_bits=34  bin_pt=0  opselect=C  inp2=PCIN>>17  opr=+  inp1=P  carry=CIN  iostate=0  explicit_period=on  period=1  dbl_ovrd=off
  Convert : xbsIndex_r3/Convert  arith_type=Unsigned  n_bits=34  bin_pt=0  quantization=Truncate  overflow=Wrap  latency=0  explicit_period=on  period=1  dbl_ovrd=off  show_param=off  inserted_by_tool=off  pipeline=off
  Simulation Multiplexer : xbsIndex_r3/Simulation Multiplexer  sim_sel=1  hw_sel=2
  Simulation Multiplexer1 : xbsIndex_r3/Simulation Multiplexer  sim_sel=1  hw_sel=2
  Simulation Multiplexer2 : xbsIndex_r3/Simulation Multiplexer  sim_sel=1  hw_sel=2
  ZBT SRAM 32Bit Generation : Subsystem
  ZBT SRAM 32Bit Simulation : Subsystem
  q : Outport
  qv : Outport  Port=2
  adlocb_out : Outport  Port=3
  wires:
  Constant/1 -> Simulation Multiplexer2/1
  adlocb_in/1 -> ZBT SRAM 32Bit Generation/6(adlocb_in)
  ZBT SRAM 32Bit Generation/3(adlocb_out) -> Convert/1
  Simulation Multiplexer2/1 -> adlocb_out/1
  be/1 -> ZBT SRAM 32Bit Generation/5(be), ZBT SRAM 32Bit Simulation/5(be)
  Simulation Multiplexer/1 -> q/1
  Simulation Multiplexer1/1 -> qv/1
  ZBT SRAM 32Bit Generation/2(qv) -> Simulation Multiplexer1/2
  ZBT SRAM 32Bit Generation/1(q) -> Simulation Multiplexer/2
  ZBT SRAM 32Bit Simulation/1(q) -> Simulation Multiplexer/1
  ZBT SRAM 32Bit Simulation/2(qv) -> Simulation Multiplexer1/1
  d/1 -> ZBT SRAM 32Bit Simulation/1(d), ZBT SRAM 32Bit Generation/1(d)
  a/1 -> ZBT SRAM 32Bit Simulation/2(a), ZBT SRAM 32Bit Generation/2(a)
  w/1 -> ZBT SRAM 32Bit Simulation/3(w), ZBT SRAM 32Bit Generation/3(w)
  r/1 -> ZBT SRAM 32Bit Simulation/4(r), ZBT SRAM 32Bit Generation/4(r)
  Convert/1 -> Simulation Multiplexer2/2
